(* Logix 5000 DataType export Set_Ramp; software revision 32.01 *)

TYPE Set_Ramp :
STRUCT
   Address : SINT;   // 1-31=Address 1-31, 32-62=Address 1B-31B
   Ramp : SINT;   // 0=No Ramp, 1=50ms, 2=100ms, 3=200ms, 4=300ms, 5=500ms, 6=1s, 7=1.5s
END_STRUCT
END_TYPE
